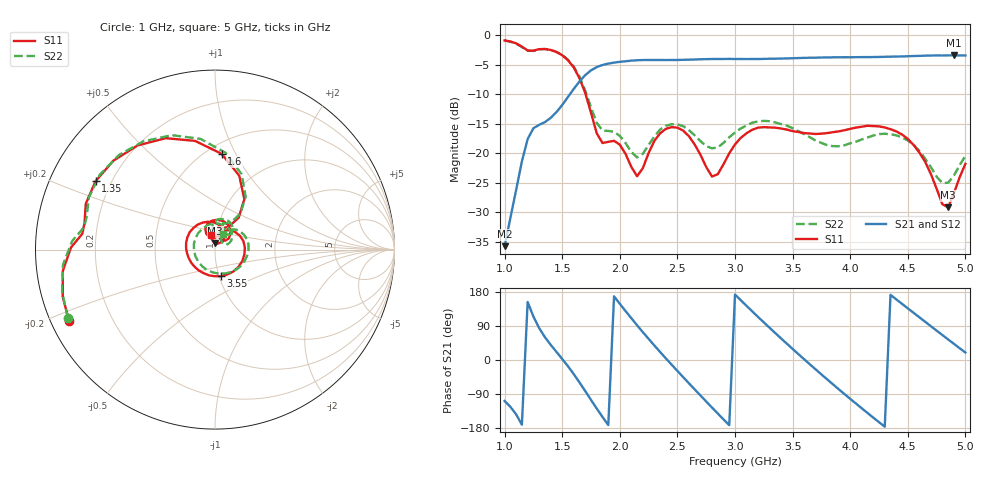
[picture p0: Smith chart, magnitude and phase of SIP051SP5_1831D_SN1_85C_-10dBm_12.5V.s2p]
# GHz  S  dB  R  50
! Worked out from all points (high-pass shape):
!   81 points, 1 GHz to 5 GHz, reference 50 ohm
!   highest |S21| = -3.39 dB at 4.9 GHz (marker M1); lowest = -35.7 dB at 1 GHz (marker M2)
!   |S21| within 3 dB of the highest: 1.722 GHz to end of sweep
!   lowest |S11| = -29.2 dB at 4.85 GHz (marker M3), VSWR 1.07, Z = 50 + j3.48 ohm
!   |S11| at or under -10 dB: 1.703 GHz to end of sweep
!   |S22| runs from -25.0 to -0.9 dB; largest |S21 - S12| = 0.0022
!   S11 on the Smith chart (normalised r, x): 1 GHz: 0.05, -0.23; 1.35 GHz: 0.14, +0.26; 1.6 GHz: 0.59, +0.88; 3.55 GHz: 1.02, -0.31; 5 GHz: 0.95, +0.15
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1  -0.86 -153.8  -35.73 -108.1  -35.45 -108.0  -0.88 -155.2
1.2  -2.57 173.2  -17.58 153.0  -17.54 152.8  -2.61 170.3
1.35  -2.30 150.2  -14.71 60.2  -14.69 60.3  -2.32 147.0
1.6  -5.43 86.1  -9.08 -37.2  -9.07 -37.2  -5.31 83.8
1.7  -9.77 59.8  -6.74 -82.0  -6.74 -82.0  -9.36 59.8
1.8  -16.60 59.1  -5.37 -128.3  -5.37 -128.2  -14.83 59.0
1.95  -17.87 80.5  -4.61 167.9  -4.62 168.0  -16.33 71.8
2.15  -23.88 95.6  -4.22 91.7  -4.22 91.8  -20.68 80.7
2.35  -16.60 106.8  -4.18 21.1  -4.16 21.1  -15.95 89.9
2.5  -15.63 73.5  -4.17 -28.9  -4.15 -28.9  -15.09 65.2
2.7  -20.23 39.0  -4.05 -93.6  -4.03 -93.5  -17.91 44.5
2.8  -23.92 51.7  -4.00 -125.4  -3.98 -125.4  -19.15 49.3
3  -18.48 62.5  -4.00 172.8  -3.99 172.8  -16.46 48.9
3.25  -15.56 4.2  -3.99 99.3  -3.98 99.3  -14.49 9.5
3.55  -16.38 -77.6  -3.84 15.6  -3.83 15.6  -16.23 -53.3
3.7  -16.71 -115.6  -3.79 -24.7  -3.77 -24.7  -17.84 -94.4
4  -15.85 177.3  -3.71 -102.4  -3.70 -102.4  -18.29 165.5
4.35  -15.90 104.6  -3.61 171.9  -3.62 171.9  -16.77 74.0
4.6  -19.85 58.4  -3.48 112.8  -3.47 112.8  -19.57 29.6
4.85  -29.17 87.4  -3.39 54.2  -3.40 54.3  -24.98 47.5
4.9  -26.77 102.8  -3.39 42.7  -3.39 42.7  -23.76 58.8
5  -21.78 104.6  -3.41 19.7  -3.41 19.7  -20.40 62.8
